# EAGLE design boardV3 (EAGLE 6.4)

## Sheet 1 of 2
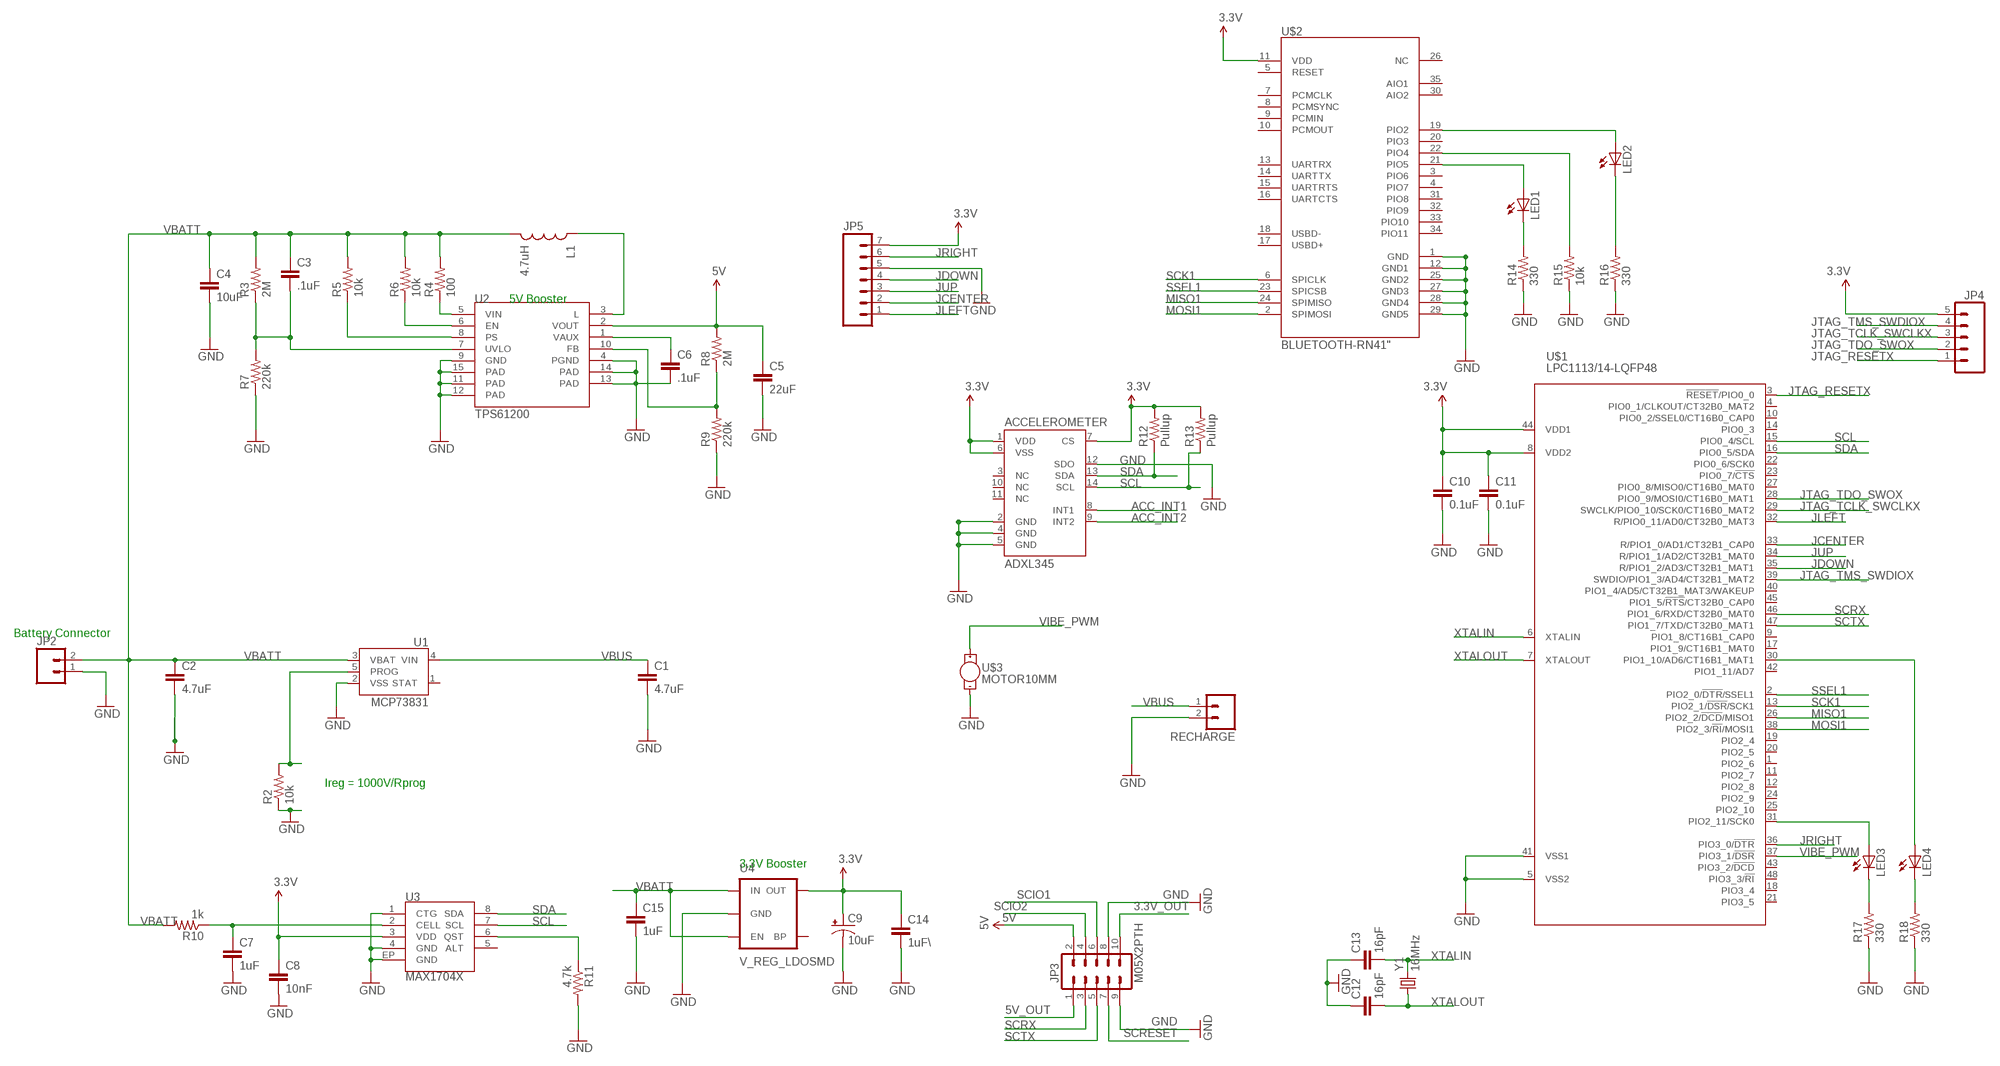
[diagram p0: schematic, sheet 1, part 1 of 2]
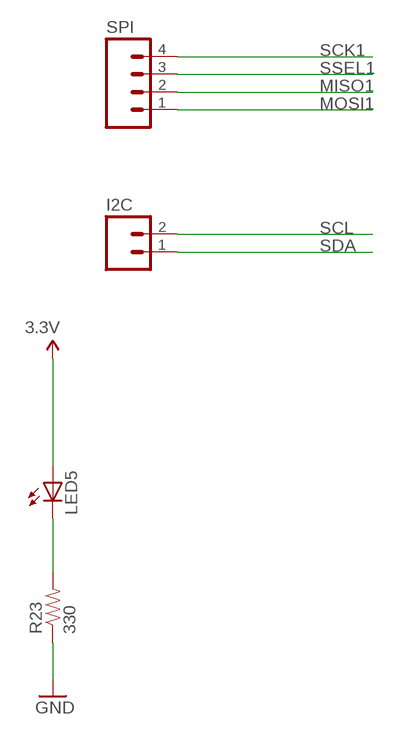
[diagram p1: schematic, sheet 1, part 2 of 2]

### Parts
ACCELEROMETER  ADXL345  [LGA14]
C1  4.7uF  CAP0603-CAP  [0603-CAP]
C2  4.7uF  CAP0603-CAP  [0603-CAP]
C3  .1uF  CAP0603-CAP  [0603-CAP]
C4  10uF  CAP0603-CAP  [0603-CAP]
C5  22uF  CAP0603-CAP  [0603-CAP]
C6  .1uF  CAP0603-CAP  [0603-CAP]
C7  1uF  CAP0603-CAP  [0603-CAP]
C8  10nF  CAP0603-CAP  [0603-CAP]
C9  10uF  10UF-TANT  [EIA3216]
C10  0.1uF  CAP0603-CAP  [0603-CAP]
C11  0.1uF  CAP0603-CAP  [0603-CAP]
C12  16pF  CAP0603-CAP  [0603-CAP]
C13  16pF  CAP0603-CAP  [0603-CAP]
C14  1uF\  CAP0603-CAP  [0603-CAP]
C15  1uF  CAP0603-CAP  [0603-CAP]
I2C  M02POLAR  [MOLEX-1X2]
JP2  M02PTH  [1X02]
JP3  M05X2PTH  [AVR_ICSP]
JP4  M05PTH  [1X05]
JP5  M07  [1X07]
L1  4.7uH  INDUCTOR.  [CDRH2D09]
LED1  LED0603  [LED-0603]
LED2  LED0603  [LED-0603]
LED3  LED0603  [LED-0603]
LED4  LED0603  [LED-0603]
LED5  LED0603  [LED-0603]
R2  10k  RESISTOR0603-RES  [0603-RES]
R3  2M  RESISTOR0603-RES  [0603-RES]
R4  100  RESISTOR0603-RES  [0603-RES]
R5  10k  RESISTOR0603-RES  [0603-RES]
R6  10k  RESISTOR0603-RES  [0603-RES]
R7  220k  RESISTOR0603-RES  [0603-RES]
R8  2M  RESISTOR0603-RES  [0603-RES]
R9  220k  RESISTOR0603-RES  [0603-RES]
R10  1k  RESISTOR0603-RES  [0603-RES]
R11  4.7k  RESISTOR0603-RES  [0603-RES]
R12  Pullup  RESISTOR0603-RES  [0603-RES]
R13  Pullup  RESISTOR0603-RES  [0603-RES]
R14  330  RESISTOR0603-RES  [0603-RES]
R15  10k  RESISTOR0603-RES  [0603-RES]
R16  330  RESISTOR0603-RES  [0603-RES]
R17  330  RESISTOR0603-RES  [0603-RES]
R18  330  RESISTOR0603-RES  [0603-RES]
R23  330  RESISTOR0603-RES  [0603-RES]
RECHARGE  M02POLAR  [MOLEX-1X2]
SPI  M04POLAR  [MOLEX-1X4]
U1  MCP73831  [SOT23-5]
U2  TPS61200  [QFN-10_PAD]
U3  MAX1704X  [TDFN-8]
U4  V_REG_LDOSMD  [SOT23-5]
U$1  LPC1113/14-LQFP48  [LQFP48]
U$2  BLUETOOTH-RN41"  [RN41]
U$3  MOTOR10MM  [VIBE-MOTOR-10MM]
Y1  16MHz  CRYSTAL5X3  [CRYSTAL-SMD-5X3]

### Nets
3.3V: ACCELEROMETER.1(VDD) ACCELEROMETER.6(VSS) ACCELEROMETER.7(CS) C8.1 C9.A(+) C10.1 C11.1 C14.1 JP4.5 JP5.7 LED5.A R12.2 R13.2 U3.3(VDD) U4.5(OUT) U$1.8(VDD2) U$1.44(VDD1) U$2.11(VDD) ; also sheet 2
3.3V_OUT: JP3.10
5V: C5.1 JP3.2 R8.2 U2.2(VOUT)
5V_OUT: JP3.1
ACC_INT1: ACCELEROMETER.8(INT1)
ACC_INT2: ACCELEROMETER.9(INT2)
GND: ACCELEROMETER.2(GND) ACCELEROMETER.4(GND) ACCELEROMETER.5(GND) ACCELEROMETER.12(SDO) C1.2 C2.2 C4.2 C5.2 C6.2 C7.2 C8.2 C9.C(-) C10.2 C11.2 C12.1 C13.1 C14.2 C15.2 JP2.1 JP3.8 JP3.9 JP5.5 R2.1 R7.1 R9.1 R11.2 R14.1 R15.1 R16.1 R17.1 R18.1 R23.1 RECHARGE.2 U1.2(VSS) U2.4(PGND) U2.9(GND) U2.11(PAD) U2.12(PAD) U2.13(PAD) U2.14(PAD) U2.15(PAD) U3.1(CTG) U3.4(GND) U3.EP(GND) U4.2(GND) U$1.5(VSS2) U$1.41(VSS1) U$2.1(GND) U$2.12(GND1) U$2.25(GND2) U$2.27(GND3) U$2.28(GND4) U$2.29(GND5) U$3.- ; also sheet 2
JCENTER: JP5.2 U$1.33(R/PIO1_0/AD1/CT32B1_CAP0) ; also sheet 2
JDOWN: JP5.4 U$1.35(R/PIO1_2/AD3/CT32B1_MAT1) ; also sheet 2
JLEFT: JP5.1 U$1.32(R/PIO0_11/AD0/CT32B0_MAT3) ; also sheet 2
JRIGHT: JP5.6 U$1.36(PIO3_0/!DTR!) ; also sheet 2
JTAG_RESETX: JP4.1 U$1.3(!RESET!/PIO0_0)
JTAG_TCLK_SWCLKX: JP4.3 U$1.29(SWCLK/PIO0_10/SCK0/CT16B0_MAT2)
JTAG_TDO_SWOX: JP4.2 U$1.28(PIO0_9/MOSI0/CT16B0_MAT1)
JTAG_TMS_SWDIOX: JP4.4 U$1.39(SWDIO/PIO1_3/AD4/CT32B1_MAT2)
JUP: JP5.3 U$1.34(R/PIO1_1/AD2/CT32B1_MAT0) ; also sheet 2
MISO1: SPI.2 U$1.26(PIO2_2/!DCD!/MISO1) U$2.24(SPIMISO)
MOSI1: SPI.1 U$1.38(PIO2_3/!RI!/MOSI1) U$2.2(SPIMOSI)
N$1: LED2.A U$2.19(PIO2)
N$2: R2.2 U1.5(PROG)
N$3: C3.2 R3.1 R7.2 U2.7(UVLO)
N$4: C6.1 U2.1(VAUX)
N$5: R6.1 U2.6(EN)
N$6: R5.1 U2.8(PS)
N$7: L1.P$1 U2.3(L)
N$8: R8.1 R9.2 U2.10(FB)
N$9: C7.1 R10.1 U3.2(CELL)
N$10: R11.1 U3.6(QST)
N$11: R15.2 U$2.22(PIO4)
N$12: LED1.A U$2.21(PIO5)
N$13: LED1.C R14.2
N$14: LED2.C R16.2
N$15: LED3.A U$1.31(PIO2_11/SCK0)
N$16: LED4.A U$1.30(PIO1_10/AD6/CT16B1_MAT1)
N$17: LED3.C R17.2
N$18: LED4.C R18.2
N$21: LED5.C R23.2
SCIO1: JP3.6
SCIO2: JP3.4
SCK1: SPI.4 U$1.13(PIO2_1/!DSR!/SCK1) U$2.6(SPICLK)
SCL: ACCELEROMETER.14(SCL) I2C.2 R13.1 U3.7(SCL) U$1.15(PIO0_4/SCL)
SCRESET: JP3.7
SCRX: JP3.3 U$1.46(PIO1_6/RXD/CT32B0_MAT0)
SCTX: JP3.5 U$1.47(PIO1_7/TXD/CT32B0_MAT1)
SDA: ACCELEROMETER.13(SDA) I2C.1 R12.1 U3.8(SDA) U$1.16(PIO0_5/SDA)
SSEL1: SPI.3 U$1.2(PIO2_0/!DTR!/SSEL1) U$2.23(SPICSB)
VBATT: C2.1 C3.1 C4.1 C15.1 JP2.2 L1.P$2 R3.2 R4.2 R5.2 R6.2 R10.2 U1.3(VBAT) U4.1(IN) U4.3(EN)
VBUS: C1.1 RECHARGE.1 U1.4(VIN)
VIBE_PWM: U$1.37(PIO3_1/!DSR!) U$3.+
VIN: R4.1 U2.5(VIN)
XTALIN: C13.2 U$1.6(XTALIN) Y1.3
XTALOUT: C12.2 U$1.7(XTALOUT) Y1.1
Unconnected: ACCELEROMETER.3(NC) ACCELEROMETER.10(NC) ACCELEROMETER.11(NC) U1.1(STAT) U3.5(ALT) U4.4(BP) U$1.1(PIO2_6) U$1.4(PIO0_1/CLKOUT/CT32B0_MAT2) U$1.9(PIO1_8/CT16B1_CAP0) U$1.10(PIO0_2/SSEL0/CT16B0_CAP0) U$1.11(PIO2_7) U$1.12(PIO2_8) U$1.14(PIO0_3) U$1.17(PIO1_9/CT16B1_MAT0) U$1.18(PIO3_4) U$1.19(PIO2_4) U$1.20(PIO2_5) U$1.21(PIO3_5) U$1.22(PIO0_6/SCK0) U$1.23(PIO0_7/!CTS!) U$1.24(PIO2_9) U$1.25(PIO2_10) U$1.27(PIO0_8/MISO0/CT16B0_MAT0) U$1.40(PIO1_4/AD5/CT32B1_MAT3/WAKEUP) U$1.42(PIO1_11/AD7) U$1.43(PIO3_2/!DCD!) U$1.45(PIO1_5/!RTS!/CT32B0_CAP0) U$1.48(PIO3_3/!RI!) U$2.3(PIO6) U$2.4(PIO7) U$2.5(RESET) U$2.7(PCMCLK) U$2.8(PCMSYNC) U$2.9(PCMIN) U$2.10(PCMOUT) U$2.13(UARTRX) U$2.14(UARTTX) U$2.15(UARTRTS) U$2.16(UARTCTS) U$2.17(USBD+) U$2.18(USBD-) U$2.20(PIO3) U$2.26(NC) U$2.30(AIO2) U$2.31(PIO8) U$2.32(PIO9) U$2.33(PIO10) U$2.34(PIO11) U$2.35(AIO1)

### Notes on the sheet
- 5V Booster
- Battery Connector
- Ireg = 1000V/Rprog
- 3.3V Booster

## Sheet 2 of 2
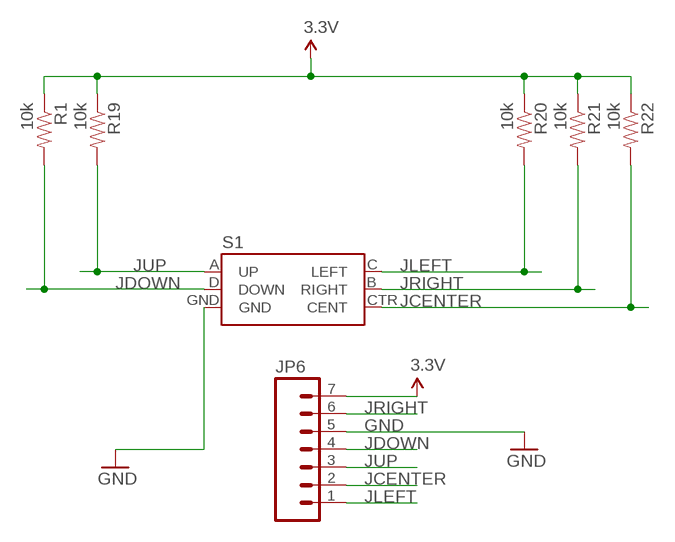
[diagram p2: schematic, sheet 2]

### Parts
JP6  M07  [1X07]
R1  10k  RESISTOR0603-RES  [0603-RES]
R19  10k  RESISTOR0603-RES  [0603-RES]
R20  10k  RESISTOR0603-RES  [0603-RES]
R21  10k  RESISTOR0603-RES  [0603-RES]
R22  10k  RESISTOR0603-RES  [0603-RES]
S1  JOYSTICK_MINI  [JOYSTICK_MINI]

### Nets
3.3V: JP6.7 R1.1 R19.1 R20.1 R21.1 R22.1 ; also sheet 1
GND: JP6.5 S1.GND ; also sheet 1
JCENTER: JP6.2 R22.2 S1.CTR(CENT) ; also sheet 1
JDOWN: JP6.4 R1.2 S1.D(DOWN) ; also sheet 1
JLEFT: JP6.1 R20.2 S1.C(LEFT) ; also sheet 1
JRIGHT: JP6.6 R21.2 S1.B(RIGHT) ; also sheet 1
JUP: JP6.3 R19.2 S1.A(UP) ; also sheet 1

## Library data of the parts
ACCELEROMETER = SparkFun-Sensors:ADXL345: 3-axis SPI/I2C 2/4/8/16g accelerometer
C1-C8 C10-C15 = SparkFun-Passives:CAP: Capacitor
C9 = SparkFun-Capacitors:10UF-TANT: 10uF Tantalum SMT; PROD_ID: CAP-00811
I2C JP2 RECHARGE = SparkFun-Connectors:M02: Header 2
JP3 = SparkFun-Connectors:M05X2: Header 5x2 Standard 10-pin dual row 0.1" header. Commonly used with AVR-ISP. Use with Spark Fun Electronics SKU: PRT-00778
JP4 = SparkFun-Connectors:M05: Header 5 Standard 5-pin 0.1" header. Use with straight break away headers (SKU : PRT-00116), right angle break away headers (PRT-00553), swiss pins (PRT-00743), machine pins (PRT-00117), and female headers (PRT-00115). Molex polarized connector foot print use with SKU : PRT-08230 with associated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
JP5 JP6 = SparkFun-Connectors:M07: Header 7 Standard 7-pin 0.1" header. Use with straight break away headers (SKU : PRT-00116), right angle break away headers (PRT-00553), swiss pins (PRT-00743), machine pins (PRT-00117), and female headers (PRT-00115). NOTES ON THE VARIANTS LOCK and LOCK_LONGPADS... This footprint was designed to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
L1 = SparkFun-Passives:INDUCTOR: Inductors
LED1-LED5 = SparkFun-LED:LED: LEDs
R1 R8 R9 R12 R13 R19-R22 = SparkFun-Resistors:RESISTOR: Resistor
R2-R7 R10 R11 R14-R18 R23 = SparkFun-Passives:RESISTOR: Resistor
S1 = SparkFun-Electromechanical:JOYSTICK_MINI: Small 5-way tactile joystick, COM-10063 4UCON SF303GJ26
SPI = SparkFun-Connectors:M04: Header 4 Standard 4-pin 0.1" header. Use with straight break away headers (SKU : PRT-00116), right angle break away headers (PRT-00553), swiss pins (PRT-00743), machine pins (PRT-00117), and female headers (PRT-00115). Molex polarized connector foot print use with SKU : PRT-08231 with associated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
U1 = SparkFun-PowerIC:MCP73831: Miniature single cell, fully integrated Li-Ion, Li-polymer charge management controller http://ww1.microchip.com/downloads/en/DeviceDoc/21984a.pdf IC-09995; PROD_ID: IC-09995
U2 = SparkFun-PowerIC:TPS61200: DC to DC Booster IC-10035; PROD_ID: IC-10035
U3 = SparkFun-PowerIC:MAX1704X: MAX17043/MAX17044: Battery Fuel Guage (43 is 1cell, 44 is 2cell)
U4 = SparkFun-PowerIC:V_REG_LDO: Voltage Regulator LDO Standard 150mA LDO voltage regulator in SOT-23 layout. Micrel part MIC5205. BP (by-pass) pin is used to lower output noise with 470pF cap.
U$1 = lpc1100v1.1:LPC1113/14-LQFP48: NXP Semiconductors LPC11xx microcontrollers ARM 32-bit Cortex-M0 Microcontroller with MPU CPU clock up to 50MHz Up to 32KByte on-chip Flash ROM with In-System Programming (ISP) and In-Application Programming (IAP) via On-Chip Bootloader Up to 8KByte SRAM Nested Vectored Interrupt Controller Up to 2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
U$2 = SparkFun-RF:BLUETOOTH-RN41: Bluetooth SMD module
U$3 = SparkFun-Electromechanical:MOTOR: Vibration Motor- ROB-08449
Y1 = SparkFun-FreqCtrl:CRYSTAL: Various standard crystals. Proven footprints. Spark Fun Electronics SKU : COM-00534

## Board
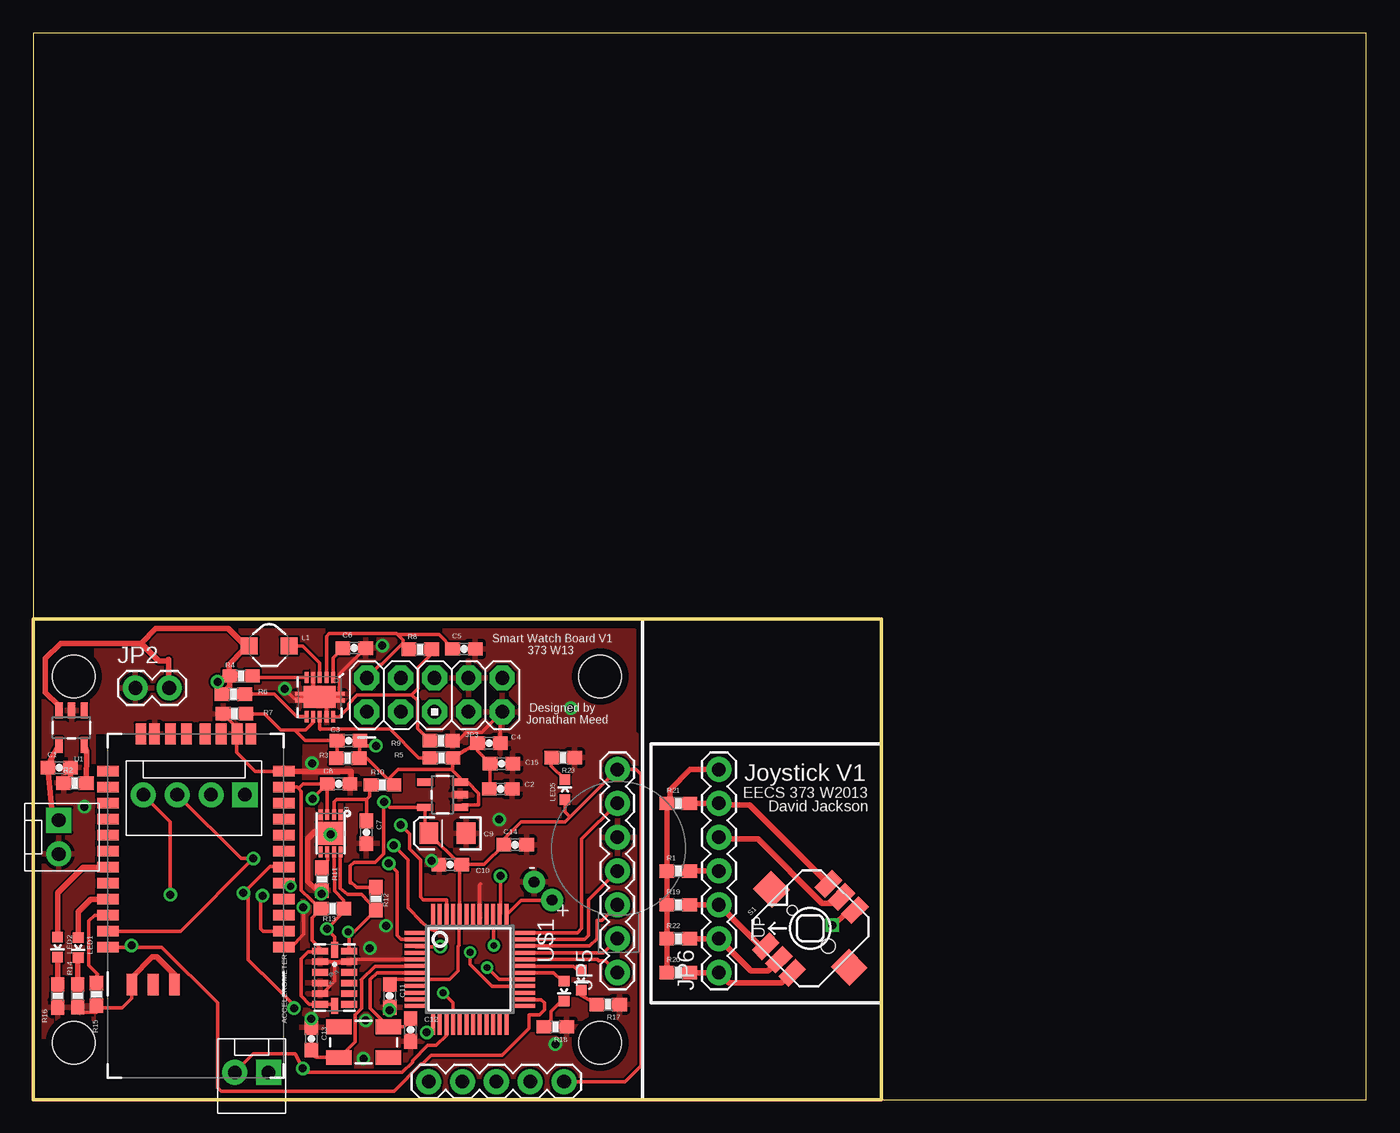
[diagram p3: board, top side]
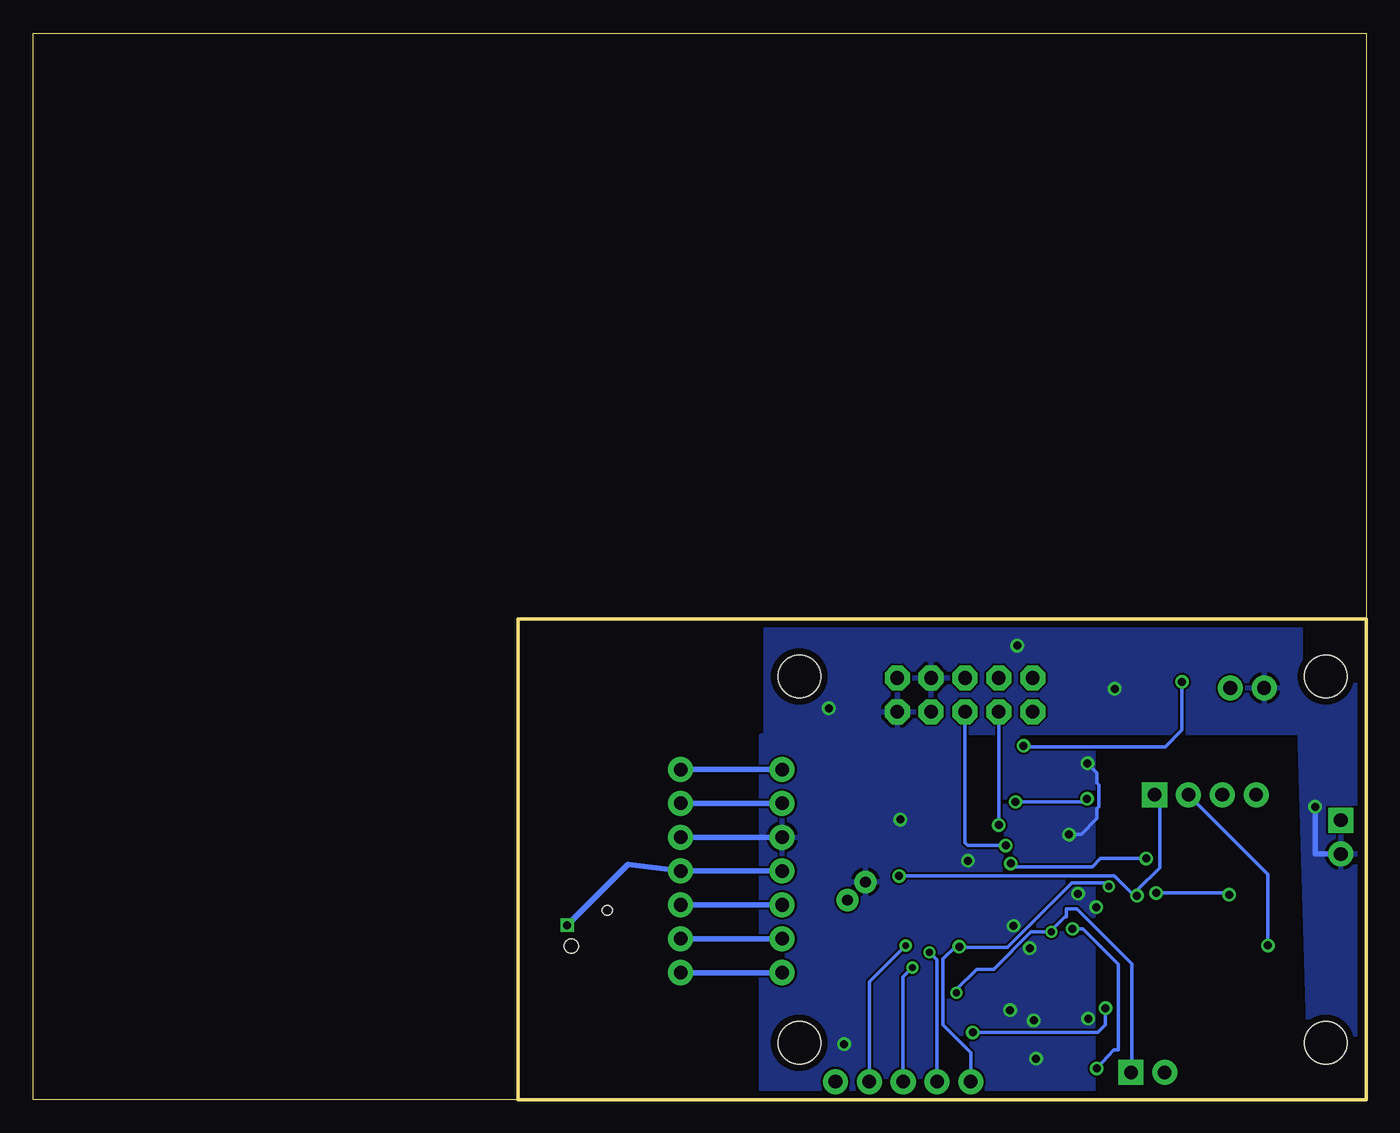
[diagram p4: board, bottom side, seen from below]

Size 100 x 80 mm. Coordinates in mm from the lower left corner, seen from the top.
Outline: 63.5,0 63.47,0 0,0 0,36.07
Outline: 63.5,0 100,0 100,80 0,80 0,36.07
Outline: 0,36.07 63.47,36.07
Outline: 63.5,0 63.63,0 63.63,36.07
Copper layers (1*16): Top 0.0178mm / dielectric 59mil / Bottom 0.0178mm
Design rules "default": minimum track width 6mil, minimum drill 14mil, track to track 6mil, track to pad 6mil, pad to pad 6mil, via to via 6mil, smd to smd 6mil, copper to edge 20mil, drill to drill 16mil, minimum pad ring 8mil, minimum via ring 8mil, stop-mask expansion 3mil, vias tented up to drill 0mil, thermal gap 10mil
Holes 3.2 mm at 42.53,31.75 3.03,31.75 3.03,4.25 42.53,4.25

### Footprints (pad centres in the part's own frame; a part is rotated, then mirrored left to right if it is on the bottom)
LGA14 = smd 0.5 x 1.2: 1 2,1.1; 2 1.2,1.1; 3 0.4,1.1; 4 -0.4,1.1; 5 -1.2,1.1; 6 -2,1.1; 8 -2,-1.1; 9 -1.2,-1.1; 10 -0.4,-1.1; 11 0.4,-1.1; 12 1.2,-1.1; 13 2,-1.1 | smd 1.2 x 0.5: 7 -2.1,0; 14 2.1,0
0603-CAP = smd 1.1 x 1: 1 -0.85,0; 2 0.85,0
EIA3216 = smd 1.4 x 1.6: A 1.4,0; C -1.4,0
MOLEX-1X2 = drill 1.016 pad 1.88 square: 1 0,0 | drill 1.016 pad 1.88: 2 2.54,0
1X02 = drill 1.016 pad 1.88: 1 0,0; 2 2.54,0
AVR_ICSP = drill 1.016 pad 1.88 octagon: 1 -1.27,5.08; 2 1.27,5.08; 3 -1.27,2.54; 4 1.27,2.54; 5 -1.27,0; 6 1.27,0; 7 -1.27,-2.54; 8 1.27,-2.54; 9 -1.27,-5.08; 10 1.27,-5.08
1X05 = drill 1.016 pad 1.88: 1 0,0; 2 2.54,0; 3 5.08,0; 4 7.62,0; 5 10.16,0
1X07 = drill 1.016 pad 1.88: 1 0,0; 2 2.54,0; 3 5.08,0; 4 7.62,0; 5 10.16,0; 6 12.7,0; 7 15.24,0
CDRH2D09 = smd 1.3 x 1.3: P$1 -1.5,0; P$2 1.5,0
LED-0603 = smd 0.8 x 0.8: A 0,-0.75; C 0,0.75
0603-RES = smd 1.1 x 1: 1 -0.85,0; 2 0.85,0
JOYSTICK_MINI = smd 1.85 x 1.1: A -3.325,1.4; B 3.325,1.4; C -3.325,-1.4; CTR -3.325,0; D 3.325,-1.4; GND 3.325,0 | smd 1.9 x 2: NC 0,4.13; NC@0 0,-4.13 | hole 0.75: 0,1.9 | hole 1.05: 0,-1.9
MOLEX-1X4 = drill 1.016 pad 1.88 square: 1 0,0 | drill 1.016 pad 1.88: 2 2.54,0; 3 5.08,0; 4 7.62,0
SOT23-5 = smd 0.55 x 1.2: 1 -0.95,-1.3; 2 0,-1.3; 3 0.95,-1.3; 4 0.95,1.3; 5 -0.95,1.3
QFN-10_PAD = smd 0.297 x 0.85: 1 -1,-1.475; 2 -0.5,-1.475; 3 0,-1.475; 4 0.5,-1.475; 5 1,-1.475; 6 1,1.475; 7 0.5,1.475; 8 0,1.475; 9 -0.5,1.475; 10 -1,1.475 | smd 0.7 x 0.28: 11 -1.5,0.25; 12 -1.5,-0.25; 13 1.5,0.25; 14 1.5,-0.25 | smd 2.4 x 1.65: 15 0,0
TDFN-8 = smd 0.8 x 0.3: 1 -1.4,0.75; 2 -1.4,0.25; 3 -1.4,-0.25; 4 -1.4,-0.75; 5 1.4,-0.75; 6 1.4,-0.25; 7 1.4,0.25; 8 1.4,0.75 | smd 1.73 x 1.88: EP 0,0
LQFP48 = smd 0.3 x 1.6: 1 -2.75,-4.1; 2 -2.25,-4.1; 3 -1.75,-4.1; 4 -1.25,-4.1; 5 -0.75,-4.1; 6 -0.25,-4.1; 7 0.25,-4.1; 8 0.75,-4.1; 9 1.25,-4.1; 10 1.75,-4.1; 11 2.25,-4.1; 12 2.75,-4.1; 25 2.75,4.1; 26 2.25,4.1; 27 1.75,4.1; 28 1.25,4.1; 29 0.75,4.1; 30 0.25,4.1; 31 -0.25,4.1; 32 -0.75,4.1; 33 -1.25,4.1; 34 -1.75,4.1; 35 -2.25,4.1; 36 -2.75,4.1 | smd 1.6 x 0.3: 13 4.1,-2.75; 14 4.1,-2.25; 15 4.1,-1.75; 16 4.1,-1.25; 17 4.1,-0.75; 18 4.1,-0.25; 19 4.1,0.25; 20 4.1,0.75; 21 4.1,1.25; 22 4.1,1.75; 23 4.1,2.25; 24 4.1,2.75; 37 -4.1,2.75; 38 -4.1,2.25; 39 -4.1,1.75; 40 -4.1,1.25; 41 -4.1,0.75; 42 -4.1,0.25; 43 -4.1,-0.25; 44 -4.1,-0.75; 45 -4.1,-1.25; 46 -4.1,-1.75; 47 -4.1,-2.25; 48 -4.1,-2.75
RN41 = smd 0.8 x 1.6: 1 -6.6,-6.6; 2 -5.4,-6.6; 3 -4.2,-6.6; 4 -3,-6.6; 5 -1.8,-6.6; 6 -0.6,-6.6; 7 0.6,-6.6; 8 1.8,-6.6; 9 3,-6.6; 10 4.2,-6.6; 11 5.4,-6.6; 12 6.6,-6.6; 13 6.6,6.6; 14 5.4,6.6; 15 4.2,6.6; 16 3,6.6; 17 1.8,6.6; 18 0.6,6.6; 19 -0.6,6.6; 20 -1.8,6.6; 21 -3,6.6; 22 -4.2,6.6; 23 -5.4,6.6; 24 -6.6,6.6 | smd 1.6 x 0.8: 25 -9.4,4.8; 26 -9.4,3.2; 27 -9.4,1.6; 28 9.4,3.1; 29 9.4,-3.1; 30 9.4,-4.122; 31 9.4,-1.9; 32 9.4,-0.7; 33 9.4,0.7; 34 9.4,1.9; 35 9.4,4.122
VIBE-MOTOR-10MM = drill 0.8 pad 1.676: + -5,-3.9; - -6.35,-2.54
CRYSTAL-SMD-5X3 = smd 1.9 x 1.1: 1 -1.85,-1.15; 2 1.85,-1.15; 3 1.85,1.15; 4 -1.85,1.15

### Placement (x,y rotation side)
ACCELEROMETER  22.61,9.15 90 top
C1  1.95,24.9 0 top
C2  35.07,23.3 0 top
C3  23.64,26.93 180 top
C4  34.18,26.73 0 top
C5  32.31,33.8 0 top
C6  24.09,33.87 0 top
C7  24.98,20.06 270 top
C8  22.9,23.68 0 top
C9  31.07,19.98 180 top
C10  31.28,17.63 180 top
C11  26.74,7.77 270 top
C12  28.3,5.22 90 top
C13  20.87,4.57 270 top
C14  36.16,19.11 0 top
C15  35.12,25.2 0 top
I2C  17.65,2.03 180 top
JP2  7.65,30.88 0 top
JP3  30.1,30.36 90 top
JP4  29.66,1.35 0 top
JP5  43.81,9.53 90 top
JP6  51.44,9.53 90 top
L1  17.69,34.03 180 top
LED1  3.36,11.41 180 top
LED2  1.82,11.44 180 top
LED3  41.1,8.97 180 top
LED4  39.82,8.14 180 top
LED5  39.88,23.24 0 top
R1  48.39,17.14 0 top
R2  3.12,23.74 0 top
R3  23.59,25.61 0 top
R4  15.59,31.78 180 top
R5  30.62,25.63 0 top
R6  15.01,30.41 180 top
R7  15.09,28.94 0 top
R8  29.03,33.78 180 top
R9  30.59,26.92 180 top
R10  26.19,23.6 0 top
R11  21.66,16.53 270 top
R12  25.71,15.06 90 top
R13  22.45,14.32 180 top
R14  3.33,7.79 90 top
R15  4.74,7.9 90 top
R16  1.83,7.77 90 top
R17  43.13,7.13 180 top
R18  39.17,5.46 180 top
R19  48.39,14.61 0 top
R20  48.39,9.53 0 top
R21  48.39,22.23 0 top
R22  48.39,12.06 0 top
R23  39.75,25.65 180 top
RECHARGE  1.91,20.95 270 top
S1  58.29,12.85 45 top
SPI  15.88,22.86 180 top
U1  2.86,27.9 180 top
U2  21.49,30.19 180 top
U3  22.31,19.98 270 top
U4  30.71,22.87 90 top
U$1  32.74,9.76 270 top
U$2  12.19,18.03 90 top
U$3  43.92,18.86 0 top
Y1  24.78,4.31 180 top

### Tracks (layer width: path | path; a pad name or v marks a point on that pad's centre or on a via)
3.3V  (via drill 0.6)
  Top 0.254: ACCELEROMETER.7 22.51,7.14 ACCELEROMETER.6 20.7,7.14 20.08,7.77 20.08,10.54 20.61,11.06 21.43,11.06 ACCELEROMETER.1 | ACCELEROMETER.1 21.51,11.06 21.55,11.01 | ACCELEROMETER.1 21.51,11.35 20.92,11.94 20.92,13.65 R13.2 21.48,14.32 20.79,15.02 | 19.89,23.34 20.11,23.13 20.11,15.7 20.79,15.02 | 19.89,23.34 19.79,23.45 18.81,23.45 U$2.11 | C8.1 U3.3 | C8.1 20.23,23.68 19.89,23.34 | v20.95,22.57 v20.95,22.58 C8.1 | C9.A 29.41,20.24 U4.5 26.72,21.92 v26.31,22.33 26.27,22.29 26.27,18.42 25.64,17.79 24.06,17.79 23.79,17.52 23.79,16.38 | 30,19.65 C9.A | C10.1 32.2,17.63 | 32.2,17.63 32.2,17.62 | C10.1 32.02,17.63 C9.A | 23.79,16.26 23.79,16.38 | C11.1 27.13,9.01 U$1.8 31.24,9.01 31.88,9.65 31.88,11.5 31.95,11.57 31.95,13.82 U$1.44 31.99,17.49 C10.1 | 32.2,17.63 33.82,17.63 C14.1 35.31,19.56 36.58,20.83 39.88,20.83 40.26,21.21 | 40.26,21.21 JP5.7 45.21,24.77 45.59,24.38 45.59,2.54 44.4,1.35 JP4.5 | LED5.A 39.88,21.59 40.26,21.21 | 20.79,15.02 | R12.2 24.25,15.91 23.79,16.38
  Top 0.406: JP6.7 49.28,24.77 47.75,23.24 47.75,22.44 R21.1 R1.1 R19.1 R22.1 R20.1
  Bottom 0.254: v26.31,22.33 21.18,22.33 v20.95,22.57
  Bottom 0.406: JP5.7 JP6.7
5V
  Top 0.254: U2.2 21.99,34.76 22.2,34.97 27.27,34.97 27.38,34.85 | 27.38,34.85 27.75,34.48 27.75,34.27 27.59,34.11 | 27.59,34.11 26.12,32.64 26.03,32.64 JP3.2 | R8.2 27.93,33.78 27.59,34.11 | C5.1 31.46,33.86 30.44,34.88 27.41,34.88 27.38,34.85
GND  (via drill 0.6)
  Top 0.254: ACCELEROMETER.5 21.67,7.95 22.61,8.88 22.61,10.14 22.71,10.25 23.61,10.25 ACCELEROMETER.12 | ACCELEROMETER.12 ACCELEROMETER.2 | 18.79,25.01 U$2.12 16.64,24.63 15.24,26.04 15.24,27.38 U$2.29 15.53,27.68 15.51,27.68 R7.1 | U$1.5 23.88,10.51 ACCELEROMETER.12 | U$2.25 7.39,7.59 6.67,6.87 4.92,6.87 R15.1 4.74,6.54 3.33,6.54 R14.1 3.65,6.62 | U$2.1 19.34,11.43 20.29,12.38 20.29,14.38 v20.25,14.43 | 33.49,13.75 U$1.41 33.49,16.11 33.54,16.16 | 33.49,13.75 33.51,13.73 | 33.49,13.75 33.49,13.69 33.55,13.63 | U2.12 22.99,31.93 C6.2 | C4.2 35.03,28.94 JP3.9 33.65,27.56 32.48,27.56 31.84,26.92 R9.1 | U2.4 20.99,30.69 | U2.9 21.99,29.95 21.84,30.1 19.56,30.1 18.92,30.73 18.8,30.73 | C11.2 26.74,6.72 v26.72,6.7
  Top 0.406: U$2.25 7.39,9.14 8.94,10.69 9.26,10.69 10.63,9.32 10.63,8.68 U$2.27 | 3.44,7.03 R14.1 | C1.2 2.75,23.78 R2.1 | U$2.12 23.82,24.63 23.83,24.63 23.83,23.76 C8.2 | 20.99,30.69 U2.15 | U2.15 20.24,30.19 U2.13 | U2.15 22.74,30.19 U2.12 | JP6.5 51.44,19.56 54.36,19.56 59.18,14.73 60.18,14.73 S1.GND | R11.2 21.28,15.68 20.57,16.38 20.57,19.56 21.14,20.13 22.16,20.13 U3.EP
  Bottom 0.254: v22.3,19.89 21.39,19.89 20.19,21.08 20.19,21.84 20.07,21.97 20.07,23.62 20.19,23.75 20.19,24.51 v20.9,25.22
  Bottom 0.406: JP5.5 JP6.5 | RECHARGE.2 3.83,18.41 v3.83,21.97
  other vias: 26.45,13.03 40.32,29.35 20.86,6.06 24.77,3.07 24.94,5.94 25.25,11.36 26.18,34.05 29.88,17.92 34.96,21.01 18.87,30.81 39.16,4.16 21.63,15.45
  pour Bottom: 4.94,35.45 45.05,35.45 45.05,27.55 4.94,27.55 4.94,32.8
  pour Top: 4.81,35.21 45.03,35.21 45.03,27.61 4.58,27.61
  pour Top: 0.45,35.3 4.49,35.3 4.49,0.4 0.58,0.4 0.58,1.35
  pour Top: 20.4,27.34 45.21,27.34 45.21,0.81 20.09,0.81 20.09,2.47
  pour Bottom: 0.47,35.61 5.19,35.61 4.16,0.31 0.62,0.31 0.62,0.52
  pour Bottom: 20.58,27.29 45.36,27.29 45.36,0.31 21.61,0.31 21.61,0.57 20.52,0.57 20.52,27.24
JCENTER
  Top 0.254: U$1.33 42.76,11.01 JP5.2
  Top 0.406: R22.2 JP6.2 53.85,9.65 55.12,9.65 55.94,10.48 S1.CTR
  Bottom 0.406: JP5.2 JP6.2
JDOWN  (via drill 0.6)
  Top 0.254: U$1.35 41.35,12.01 41.66,12.32 41.66,14.99 JP5.4
  Top 0.406: S1.D 61.61,14.21 61.59,14.22 61.34,14.22 v59.94,13.08 | JP6.4 R1.2
  Bottom 0.406: v59.94,13.08 55.37,17.65 JP6.4 JP5.4
JLEFT
  Top 0.254: U$1.32 42.32,10.51 42.42,10.41 42.93,10.41 JP5.1
  Top 0.406: R20.2 JP6.1 52.2,8.76 56.13,8.76 56.88,9.5 S1.C
  Bottom 0.406: JP5.1 JP6.1
JRIGHT
  Top 0.254: U$1.36 40.84,12.51 41.15,12.83 41.15,19.56 JP5.6
  Top 0.406: R21.2 JP6.6 51.56,22.1 53.74,22.1 S1.B
  Bottom 0.406: JP5.6 JP6.6
JTAG_RESETX  (via drill 0.51, 0.6)
  Top 0.254: v30.53,11.47 28.68,11.47 U$1.3 | 19.07,16.23 v19.3,16
  Bottom 0.254: JP4.1 29.66,3.5 31.75,5.59 31.75,10.54 30.82,11.47 v30.53,11.47 30.49,11.43 26.92,11.43 22.1,16.26 19.56,16.26 v19.3,16
JTAG_TCLK_SWCLKX  (via drill 0.51)
  Top 0.254: v34.04,9.91 34.92,9.02 U$1.29
  Bottom 0.254: JP4.3 34.74,9.2 v34.04,9.91
JTAG_TDO_SWOX  (via drill 0.51)
  Top 0.254: v32.77,11.05 32.77,10.16 34.42,8.51 U$1.28
  Bottom 0.254: JP4.2 32.2,10.48 v32.77,11.05
JTAG_TMS_SWDIOX  (via drill 0.51)
  Top 0.254: v34.54,11.56 34.54,13.81 U$1.39
  Bottom 0.254: JP4.4 37.28,8.82 v34.54,11.56
JUP
  Top 0.254: U$1.34 41.74,11.51 42.29,12.06 42.29,13.46 42.67,13.46 JP5.3
  Top 0.406: R19.2 JP6.3 54.56,11.48 S1.A
  Bottom 0.406: JP5.3 JP6.3
MISO1  (via drill 0.6)
  Top 0.254: U$1.26 36.86,7.49 38.1,7.49 38.35,7.24 38.35,6.73 37.97,6.35 37.21,6.35 37.21,5.33 35.18,3.3 29.84,3.3 29.21,2.67 29.08,2.67 27.05,0.64 14.1,0.64 13.84,0.89 13.84,7.24 9.65,11.43 7.49,11.43 | U$2.24 7.49,11.43 | 7.49,11.43 v7.37,11.56
  Bottom 0.254: v7.37,11.56 7.37,16.89 SPI.2
MOSI1  (via drill 0.6)
  Top 0.254: U$2.2 17.23,12.63 17.04,12.82 17.04,15.14 v17.19,15.29 | v35.05,16.78 35.05,13.92 U$1.38
  Bottom 0.254: v35.05,16.78 35.04,16.77 18.89,16.77 17.41,15.29 v17.19,15.29 17.19,15.7 15.49,17.4 15.49,22.48 SPI.1
N$1
  Top 0.406: LED2.A 1.82,15.49 3.76,17.43 U$2.19
N$2
  Top 0.406: R2.2 3.99,26.12 U1.5
N$3
  Top 0.254: R7.2 17.35,28.94 18.57,27.72 19.6,27.72 | R3.1 22.79,25.66 C3.2 20.39,26.93 19.6,27.72 | U2.7 20.99,28.29 20.42,27.72 19.6,27.72
N$4
  Top 0.254: U2.1 22.49,33.13 C6.1
N$5
  Top 0.254: R6.1 18.07,30.41 19.22,29.26 19.25,29.26 19.76,28.75 20.46,28.75 U2.6
N$6
  Top 0.254: U2.8 21.49,27.82 21.54,27.78 21.56,27.8 26.75,27.8 28.92,25.63 R5.1
N$7
  Top 0.254: L1.P$1 20.2,34.03 21.46,32.77 21.46,31.7 U2.3
N$8
  Top 0.254: U2.10 22.96,28.72 23.64,29.4 23.64,29.7 24.31,30.37 28.39,30.37 | 28.39,30.37 28.81,29.95 28.81,27.85 R9.2 | 28.39,30.37 28.88,30.85 28.88,32.43 29.88,33.43 R8.1
N$9
  Top 0.254: U3.2 22.55,22.32 22.75,22.52 24.93,22.52 | 24.93,22.52 25.02,22.43 25.02,20.95 C7.1 | 24.93,22.52 25,22.52 25.23,22.74 25.23,23.59 R10.1
N$10
  Top 0.254: R11.1 21.79,17.65 22.08,17.94 22.08,18.56 U3.6
N$11
  Top 0.254: U$2.22 4.59,13.83 4.15,13.39 4.15,10.06 4.83,9.38 4.74,9.29 R15.2
N$12
  Top 0.406: LED1.A 3.36,14.07 4.3,15.01 5.56,15.01 U$2.21
N$13
  Top 0.406: R14.2 3.33,10.62 LED1.C
N$14
  Top 0.406: R16.2 LED2.C
N$15
  Top 0.254: LED3.A 40.82,9.72 40.53,10.01 U$1.31
N$16
  Top 0.254: LED4.A 39.65,8.89 39.04,9.51 U$1.30
N$17
  Top 0.254: LED3.C 41.1,7.8 R17.2
N$18
  Top 0.254: LED4.C 39.62,7.39 38.84,6.61 38.84,5.98 R18.2
N$21
  Top 0.254: LED5.C 39.88,24 38.86,25.02 38.86,25.61 R23.2
SCK1  (via drill 0.6)
  Top 0.254: U$1.13 29.99,5.51 v29.51,5.03 | v19.55,6.85 19.55,7.09 17.15,9.48 17.13,9.48 16.13,10.48 16.13,15.84 | U$2.6 18.73,17.49 17.79,17.49 16.13,15.84 | 16.13,15.84 16.1,15.84 v15.75,15.49 | v10.29,15.37 10.29,20.83 SPI.4
  Bottom 0.254: v29.51,5.03 20.13,5.03 19.55,5.61 v19.55,6.85 | v15.75,15.49 10.41,15.49 v10.29,15.37
SCL  (via drill 0.6)
  Top 0.254: U3.7 22.59,15.65 23.3,14.95 R13.1 23.3,14.07 v22.03,12.8 22.61,12.22 ACCELEROMETER.14 | U$1.15 | 30.96,5.63 U$1.15 | I2C.2 16.51,3.43 19.64,3.43 v20.22,2.34 20.53,2.03 27.69,2.03 28.45,2.79 28.45,2.92 29.59,4.06 30.23,4.06 30.99,4.83 U$1.15
  Bottom 0.254: v22.03,12.8 21.26,12.8 18.6,10.14 18.6,3.74 18.95,3.74 v20.22,2.34
SCRX  (via drill 0.6)
  Top 0.254: U$1.46 30.99,14.99 29.26,14.99 29.05,15.21 29.05,17.99 28.23,18.81 28.23,19.93 v27.56,20.6
  Bottom 0.254: v27.56,20.6 JP3.3
SCTX  (via drill 0.6)
  Top 0.254: U$1.47 30.49,12.97 30.16,12.64 29.8,12.77 29.11,13.33 29.15,13.33 28.12,14.36 28.12,17.98 v27.05,19.05
  Bottom 0.254: v27.05,19.05 29.9,19.05 30.11,19.26 JP3.5
SDA  (via drill 0.51)
  Top 0.254: 23.68,11.17 ACCELEROMETER.13 23.71,12.49 v23.62,12.57 24.07,12.57 R12.1 24.64,15.41 23.58,15.41 23.03,15.83 23.03,18.56 U3.8 | U$1.16 31.49,7.25 v30.73,8
  Bottom 0.254: I2C.1 17.57,2.11 17.57,10.17 21.71,14.31 22.48,14.31 22.48,13.72 22.6,13.72 23.62,12.7 v23.62,12.57 25.15,12.57 27.94,9.78 29.21,9.78 30.73,8.26 v30.73,8
SSEL1  (via drill 0.6)
  Top 0.254: U$2.23 11.06,12.63 v16.5,18.07 15.58,18.07 SPI.3 | 26.67,17.58 v26.67,17.71 27.3,17.07 27.3,12.32 27.59,12.03 28.62,12.03 U$1.2
  Bottom 0.254: v16.5,18.07 19.93,18.07 20.55,17.45 26.41,17.45 v26.67,17.71
VBATT  (via drill 0.6)
  Top 0.254: 15.3,31.87 14.35,31.87 v13.81,31.34 | v25.7,26.54 24.88,26.54 C3.1 24.49,25.66 R3.2 25.03,25.61 26.62,24.02 | 26.62,24.02 R10.2 | 31.47,24.69 31.4,24.76 27.36,24.76 26.62,24.02 | 31.47,24.69 R5.2 32.44,26.22 C4.1 33.33,26.14 C15.1 34.27,23.35 C2.1 | 31.47,24.69 32.01,24.15 U4.3 32.57,23.82 33.4,22.99 33.4,22.1 32.18,22.1 U4.1
  Top 0.406: U1.3 1.91,29.55 0.91,30.55 0.91,33.1 2.05,34.24 8.08,34.24 | 8.08,34.24 9.41,32.91 10.05,32.91 10.16,33.02 10.16,30.91 JP2.2 | 15.75,34.03 L1.P$2 15.96,34.03 | 15.3,31.87 R4.2 | 8.08,34.24 9.2,35.35 14.63,35.35 15.75,34.23 15.75,34.03 | 15.75,34.03 15.75,33.73 14.68,32.66 14.68,31.84 R4.2 | R4.2 14.74,30.99 R6.2
  Bottom 0.254: v13.81,31.34 13.81,27.74 15.09,26.47 25.63,26.47 v25.7,26.54
VBUS
  Top 0.406: U1.4 1.45,25.83 C1.1 1.45,21.1 1.59,20.95 RECHARGE.1
VIBE_PWM
  Top 0.254: U$3.+ 36.59,14.96 U$1.37
VIN
  Top 0.254: U2.5 16.55,31.67
  Top 0.406: 16.55,31.67 R4.1
XTALIN
  Top 0.254: Y1.3 23.29,3.16 | U$1.6 25.63,10.01 24.58,8.96 24.64,8.91 24.64,6.86 24.13,6.35 24.13,4.32 22.97,3.16 Y1.3 | Y1.3 21.21,3.16 C13.2
XTALOUT
  Top 0.254: C12.2 28.18,5.99 28.18,5.83 27.81,5.46 26.67,5.46 | 26.67,5.46 Y1.1 | 26.67,5.46 25.27,6.86 25.27,9.02 25.78,9.53 28.63,9.53 U$1.7

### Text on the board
tNames: Smart Watch Board V1 | 373 W13 | Designed by | Jonathan Meed | Joystick V1 | EECS 373 W2013 | David Jackson

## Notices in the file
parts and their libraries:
SparkFun-Connectors: Licensing: CC v3.0 Share-Alike You are welcome to use this library for commercial purposes.
